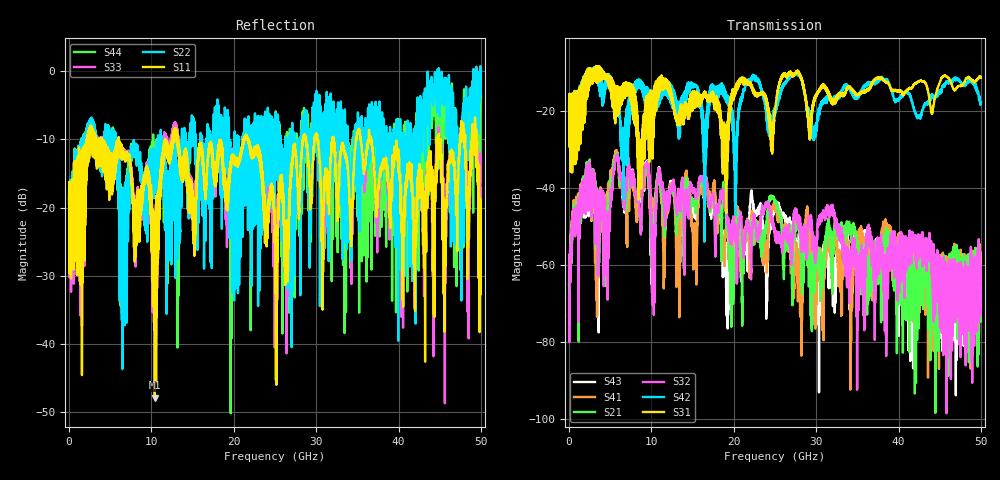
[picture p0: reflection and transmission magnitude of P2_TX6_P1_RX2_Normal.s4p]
!Keysight Technologies,N5225B,MY57041031,A.13.20.10
!Date: Friday, May 31, 2019 11:16:44
!Correction: S11(Full 4 Port(1,2,3,4))
!S12(Full 4 Port(1,2,3,4))
!S13(Full 4 Port(1,2,3,4))
!S14(Full 4 Port(1,2,3,4))
!S21(Full 4 Port(1,2,3,4))
!S22(Full 4 Port(1,2,3,4))
!S23(Full 4 Port(1,2,3,4))
!S24(Full 4 Port(1,2,3,4))
!S31(Full 4 Port(1,2,3,4))
!S32(Full 4 Port(1,2,3,4))
!S33(Full 4 Port(1,2,3,4))
!S34(Full 4 Port(1,2,3,4))
!S41(Full 4 Port(1,2,3,4))
!S42(Full 4 Port(1,2,3,4))
!S43(Full 4 Port(1,2,3,4))
!S44(Full 4 Port(1,2,3,4))
!S4P File: Measurements: <S11,S12,S13,S14>,
!<S21,S22,S23,S24>,
!<S31,S32,S33,S34>,
!<S41,S42,S43,S44>:
# Hz S  dB  R 50.0
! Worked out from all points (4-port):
!   5000 points, 10 MHz to 50 GHz, reference 50 ohm
!   strongest paths, dB at 10 MHz, 12.51 GHz, 25.01 GHz, 37.51 GHz, 50 GHz:
!     S31: -19.3, -16.8, -20.0, -11.7, -11.4
!     S42: -19.4, -16.3, -19.3, -12.4, -17.7
!     S32: -68.8, -39.7, -52.2, -54.2, -63.2
!     S21: -65.1, -40.4, -43.3, -59.2, -68.9
!     S41: -73.4, -40.0, -44.6, -58.3, -70.6
!     S43: -63.5, -39.0, -45.3, -56.6, -66.0
!   lowest |S11| = -47.8 dB at 10.41 GHz (marker M1), VSWR 1.01, Z = 50 - j0.404 ohm
!   |S11| at or under -10 dB: 13.21 GHz to 21.18 GHz (7.966 GHz wide, 46.3 % of centre); 21.74 GHz to 28.38 GHz (6.639 GHz wide, 26.5 % of centre); 36.67 GHz to 44.63 GHz (7.962 GHz wide, 19.6 % of centre)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
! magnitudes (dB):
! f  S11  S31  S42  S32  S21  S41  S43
! 10 MHz  -19.5  -19.3  -19.4  -68.8  -65.1  -73.4  -63.5
! 5.8 GHz  -13.2  -21.3  -17.8  -31.4  -30.9  -30.2  -30.7
! 10.41 GHz  -47.8  -14.9  -16.4  -57.2  -49.6  -46.7  -48.7
! 12.86 GHz  -8.3  -20.4  -19.0  -41.6  -43.2  -45.4  -43.5
! 19.21 GHz  -18.7  -24.2  -18.1  -48.1  -49.6  -49.5  -65.9
! 22.2 GHz  -12.8  -13.7  -11.2  -51.3  -51.9  -45.9  -41.4
! 50 GHz  -23.4  -11.4  -17.7  -63.2  -68.9  -70.6  -66.0
